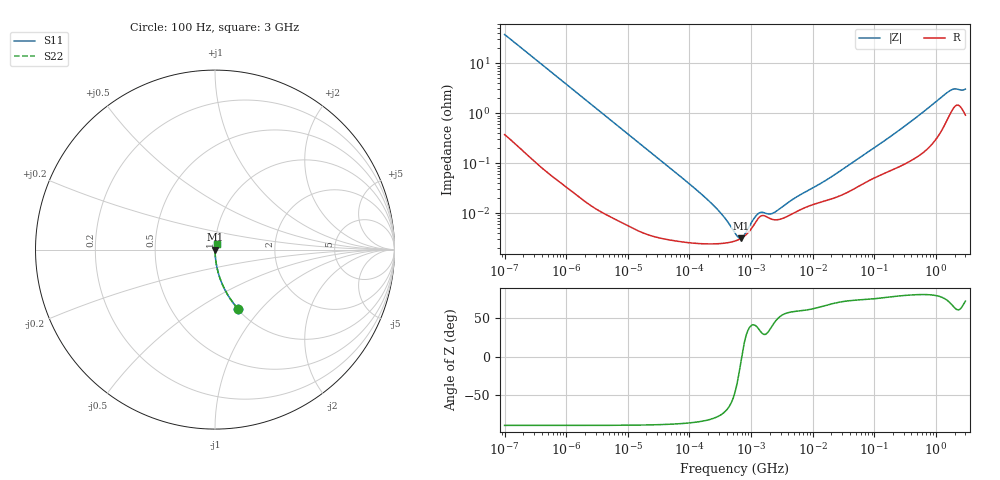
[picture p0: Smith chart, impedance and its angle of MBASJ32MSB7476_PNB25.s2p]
! MBASJ32MSB7476_PNB25  S-PARAMETER MODEL  ( Standard Model )
! Model Generated by TAIYO YUDEN Corporation (http://www.ty-top.com)
! Version 2.0
! TAIYO YUDEN Control No. 230301
! Copyright(c) 2015 TAIYO YUDEN CO.,LTD. All Rights Reserved.
! Product Description (link to TY-COMPAS)
! https://ds.yuden.co.jp/TYCOMPAS/or/detail?pn=MBASJ32MSB7476KPNB25&u=M
! Products Name : Multilayer Ceramic Capacitors
! Characteristics :
!  Capacitance : 47 [uF] , Rated Voltage : 6.3 [V] , TCC : X7R
!  Case Size : 3.2 x 2.5 / 0.126 x 0.098 [mm/inch] , Thickness : 2.5 / 0.098 [mm/inch]
!  (Conditions: Temperature = 25 [degC] , DC Bias Voltage = 0 [V])
! External Node Assignments :
!  1  o---| |---o  2
! GND o---------o GND
! Frequency Range : 100Hz  -  3GHz  [ 401 STEP ]
# MHZ S RI R 50
! Freq[MHz].  S11 Real  S11 Imag  S21 Real  S21 Imag  S12 Real  S12 Imag  S22 Real  S22 Imag
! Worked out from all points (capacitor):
!   401 points, 100 Hz to 3 GHz, reference 50 ohm
!   read as one part in series: C = 42.1 uF near 109 Hz
!   lowest |Z| = 3.13 mohm at 679.2 kHz (marker M1)
!   series resonance near 703.1 kHz, so ESL is about 1.2 nH
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0.0001  0.1272 -0.3283  0.8728 0.3283  0.8728 0.3283  0.1272 -0.3283
0.000175  0.0466 -0.2061  0.9534 0.2061  0.9534 0.2061  0.0466 -0.2061
0.000348  0.0127 -0.1077  0.9873 0.1077  0.9873 0.1077  0.0127 -0.1077
0.000724  0.00322 -0.0525  0.9968 0.0525  0.9968 0.0525  0.00322 -0.0525
0.001788  0.000651 -0.0214  0.9993 0.0214  0.9993 0.0214  0.000651 -0.0214
0.031977  3.36e-05 -0.00122  1 0.00122  1 0.00122  3.36e-05 -0.00122
0.138163  2.48e-05 -0.000274  1 0.000274  1 0.000274  2.48e-05 -0.000274
0.313007  2.46e-05 -0.000102  1 0.000102  1 0.000102  2.46e-05 -0.000102
0.35615  2.5e-05 -8.3e-05  1 8.3e-05  1 8.3e-05  2.5e-05 -8.3e-05
0.547723  2.77e-05 -2.9e-05  1 2.9e-05  1 2.9e-05  2.77e-05 -2.9e-05
0.679242  3.11e-05 -3.99e-06  1 3.99e-06  1 3.99e-06  3.11e-05 -3.99e-06
2.266852  7.45e-05 6.71e-05  0.9999 -6.71e-05  0.9999 -6.71e-05  7.45e-05 6.71e-05
2.579298  7.36e-05 8.2e-05  0.9999 -8.2e-05  0.9999 -8.2e-05  7.36e-05 8.2e-05
5.135543  0.000103 0.000173  0.9999 -0.000173  0.9999 -0.000173  0.000103 0.000173
9.794414  0.000147 0.00028  0.9999 -0.00028  0.9999 -0.00028  0.000147 0.00028
22.1892  0.000201 0.000544  0.9998 -0.000544  0.9998 -0.000544  0.000201 0.000544
175.1444  0.000701 0.00323  0.9993 -0.00323  0.9993 -0.00323  0.000701 0.00323
471.3361  0.00135 0.00803  0.9987 -0.00803  0.9987 -0.00803  0.00135 0.00803
1642.185  0.0095 0.0258  0.9905 -0.0258  0.9905 -0.0258  0.0095 0.0258
1950.712  0.0135 0.027  0.9865 -0.027  0.9865 -0.027  0.0135 0.027
2636.591  0.0128 0.0257  0.9872 -0.0257  0.9872 -0.0257  0.0128 0.0257
3000  0.00992 0.0286  0.9901 -0.0286  0.9901 -0.0286  0.00992 0.0286
